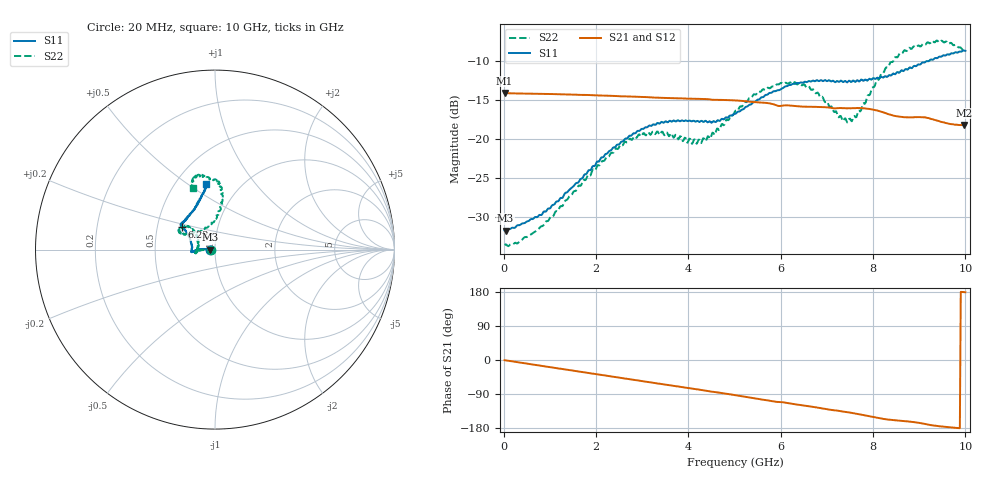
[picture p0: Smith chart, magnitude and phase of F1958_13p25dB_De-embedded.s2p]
! Integrated Device Technology
! Corporate Headquarters
! 6024 Silver Creek Valley Road
! San Jose, CA 95138  USA
! Phone:  1-408-284-8200
! Toll Free:  1-800-223-1366
! Webpage:  http://www.idt.com/
! Timing and RF Division
! 515 Groton Road, Suite 102
! Westford, MA 01886-6024
! Device:  F1958
! Description: 7-bit 0.25 dB Digital Step Attenuator
! Frequency:  0.001 -  6.000 GHz
! Package:  4x4 mm Thin QFN Plastic Package: 24 pin
! Ports:  2 RF, 12 DC
!  Pin  1  = D0
!  Pin  2  = VDD
!  Pin  3  = VMODE
!  Pin  4  = GND
!  Pin  5  = RF1  =  Port 1
!  Pin  6  = GND
!  Pin  7  = GND
!  Pin  8  = GND
!  Pin  9  = GND
!  Pin 10  = GND
!  Pin 11  = GND
!  Pin 12  = GND
!  Pin 13  = GND
!  Pin 14  = RF2  =  Port 2
!  Pin 15  = GND
!  Pin 16  = LE
!  Pin 17  = CLK
!  Pin 18  = DATA
!  Pin 19  = D6
!  Pin 20  = D5
!  Pin 21  = D4
!  Pin 22  = D3
!  Pin 23  = D2
!  Pin 24  = D1
! State:  53
! Atten State:  13.25 dB
! Voltage:  +3.30 Volts
! Current:  0.258 mA
! Data:  The device was measured on a F1958 evaluation board which has
!  individual transmission lines to the RF pins.  Data was collected
!  using a calibrated network analyzer.  The evaluation board was
!  de-embedded using Automatic Fixture Removal (AFR).
!  The reference plane is the edge of the package pin.
! Misc:
!  Action Tracker AT0419
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# GHz S dB R 50
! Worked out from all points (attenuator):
!   500 points, 20 MHz to 10 GHz, reference 50 ohm
!   highest |S21| = -14.13 dB at 20 MHz (marker M1); lowest = -18.2 dB at 9.98 GHz (marker M2)
!   lowest |S11| = -31.8 dB at 40 MHz (marker M3), VSWR 1.05, Z = 47.5 - j0.0756 ohm
!   |S11| at or under -10 dB: start of sweep to 9.212 GHz
!   |S22| runs from -33.8 to -7.4 dB; largest |S21 - S12| = 0.00053
!   S11 on the Smith chart (normalised r, x): 20 MHz: 0.95, -0.00; 6.22 GHz: 0.67, +0.18; 10 GHz: 0.70, +0.59
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0.02  -31.76 -178.2  -14.13 -0.5  -14.13 -0.5  -33.62 -177.8
0.04  -31.77 -178.2  -14.14 -0.9  -14.13 -0.9  -33.54 -176.9
0.32  -31.09 177.5  -14.18 -6.2  -14.18 -6.2  -33.32 178.9
0.72  -30.07 177.1  -14.22 -13.6  -14.21 -13.6  -31.73 179.8
1.7  -25.08 177.2  -14.36 -31.8  -14.36 -31.7  -25.61 179.8
2.6  -20.24 -179.1  -14.55 -48.3  -14.53 -48.4  -20.61 -176.0
3.36  -18.04 -174.2  -14.73 -62.4  -14.72 -62.5  -19.33 -169.1
4.26  -17.77 179.5  -14.88 -78.8  -14.90 -78.8  -20.42 167.9
4.52  -17.86 173.5  -14.99 -83.7  -15.00 -83.7  -19.21 153.5
5.02  -16.79 159.8  -15.07 -92.9  -15.08 -92.9  -16.39 139.1
5.54  -14.92 149.6  -15.32 -102.8  -15.33 -102.8  -13.93 140.3
6.22  -13.08 145.9  -15.74 -115.1  -15.75 -115.1  -12.80 151.4
6.68  -12.57 143.7  -15.89 -123.3  -15.91 -123.2  -13.69 153.4
7.3  -12.53 137.8  -16.05 -135.0  -16.06 -134.8  -17.06 132.2
7.5  -12.59 135.1  -16.09 -138.8  -16.09 -138.7  -17.41 113.9
7.68  -12.56 132.1  -16.05 -142.6  -16.05 -142.6  -16.44 97.0
8.34  -11.84 116.4  -16.85 -157.4  -16.85 -157.5  -10.66 81.6
8.68  -11.18 109.7  -17.23 -161.2  -17.23 -161.1  -8.62 86.2
9.28  -9.84 102.0  -17.49 -172.4  -17.48 -172.4  -7.42 100.4
9.68  -9.08 98.2  -18.10 -177.9  -18.13 -177.9  -7.67 106.8
9.98  -8.69 98.4  -18.24 178.9  -18.26 179.0  -8.71 109.2
10  -8.71 98.1  -18.21 178.6  -18.24 178.7  -8.79 109.4
